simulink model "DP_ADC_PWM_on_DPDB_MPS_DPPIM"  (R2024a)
settings: Solver=FixedStepDiscrete  StartTime=0.0  StopTime=inf  FixedStep=10e-6  RelTol=1e-3  EnableMultiTasking=on
model workspace (MAT data in the model file):
  Freq = 100
  Phas = 0
undefined symbols (not defined in the file): a, A0, A2, A8, AD1, AD2, AD3, AD4, AD5, ADC, address, also, AN0, AN1, AN3, AN4, as, B, B0, B5, B6, B8, below, bit, bits, BOR, C6, C7, cause, characters, Code, Communicate, contains, counter, Data, data, dead, default, deviced, disasserted, DS70005399D, dsPIC33AK512MPS506_DPDB_External_v4, dsPIC33AK512MPS506_DPDB_External_v5, dsPIC33CK64MC105, EC, ECIO, ensure, events, Family, faster, Floating, fulll, highest, HS, HS3, I, I2C, I2C1, I2C2, I2C3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
libraries: MCHP_Blockset x10, simulink x1
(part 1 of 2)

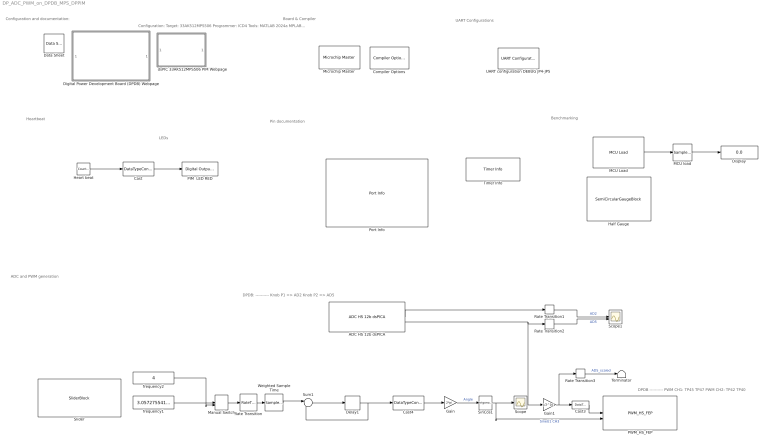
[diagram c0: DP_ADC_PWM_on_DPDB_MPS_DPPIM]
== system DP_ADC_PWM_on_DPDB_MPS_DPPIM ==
  note: DPDB: ---------- Knob P1 => AD2 Knob P2 => AD5
  note: Configuration and documentation:
  note: Configuration: Target: 33AK512MPS506 Programmer: ICD4 Tools: MATLAB 2024a MPLAB X 6.25 xc-dsc 3.21 DFP 1.2.135 MPLAB Blockset for Simulink 3.62
  note: Pin documentation
  note: Heartbeat
  note: Benchmarking
  note: ADC and PWM generation
  note: DPDB ---------- PWM CH1: TP45 TP47 PWM CH2: TP42 TP40
  note: UART Configurations
  note: LEDs
  note: Board & Compiler
  ADC HS 12b dsPICA : MCHP_Blockset/Analog IO/ADC HS 12b dsPICA  ADCREF=ADC 1 and ADC 2  ADC1_refChannel=Not used  ADC2_refChannel=0 (highest priority)  ADC3_refChannel=Not used  ADC4_refChannel=Not used  ADC5_refChannel=0 (highest priority)  CALRATE=once at startup  VREF_RNG=3.0V to 3.6V  BUFEN=on  info=0  SampleTime=10e-6  MCHP_PORT={ADC1_seq0.0}{ADC1A2}15:2:A2;{ADC2_seq0.0}{ADC2B8}15:2:B8;{ADC1_seq0.0}{ADC1A2}15:2:A2;{ADC2_seq0.0}{ADC2B8}15:2:B8;  MCHP_MASTERLINK=dsPIC33AK512MPS506_DPDB_External_v4/Microchip Master  MCHP_CRC=34143797  ADC_Synchronisation=Triggered at end of previous time step  ADC_Trig_TXT=Timer  ADC_TrigTimeStep=on  TrigSource_seq0=Dynamic Options  TrigSource_seq0_TXT=at end of previous time step  SampleTime_seq0_Tad=Dynamic Options  SampleTime_seq0_Tad_TXT="8.5 Tad  = 106ns  -  Rin < 11 kOhm"  ADC1_seq0=Dynamic Options  ADC1_seq0_TXT=AD1 AN0 / A2 / Pin[12]  ADC1_seq0_align=Left aligned  ADC1_seq0_overSampling=x1 (12 bits)  ADC2_seq0=Dynamic Options  ADC2_seq0_TXT=AD2 AN4 / B8 / Pin[23]  ADC2_seq0_align=Right aligned  ADC2_seq0_overSampling=x256 (16 bits)  ADC3_seq0=Dynamic Options  ADC3_seq0_TXT=AD3 AN1 / B5 / Pin[17]  ADC3_seq0_align=Right aligned  ADC3_seq0_overSampling=x256 (16 bits)  ADC4_seq0=Dynamic Options  ADC4_seq0_TXT=AD4 AN1 / B6 / Pin[29]  ADC4_seq0_align=Right aligned  ADC4_seq0_overSampling=x256 (16 bits)  ADC5_seq0=Dynamic Options  ADC5_seq0_TXT=AD5 AN3 / A8 / Pin[7]  ADC5_seq0_align=Right aligned  ADC5_seq0_overSampling=x256 (16 bits)  ADC1_seq0_1=Dynamic Options  ADC1_seq0_1_TXT=Not Used  ADC1_seq0_1_align=Right aligned  ADC1_seq0_1_overSampling=x1 (12 bits)  ADC2_seq0_1=Dynamic Options  ADC2_seq0_1_TXT=Not Used  ADC2_seq0_1_align=Right aligned  ADC2_seq0_1_overSampling=x1 (12 bits)  ADC3_seq0_1=Dynamic Options  ADC3_seq0_1_TXT=Not Used  ADC3_seq0_1_align=Right aligned  ADC3_seq0_1_overSampling=x1 (12 bits)  ADC4_seq0_1=Dynamic Options  ADC4_seq0_1_TXT=Not Used  ADC4_seq0_1_align=Right aligned  ADC4_seq0_1_overSampling=x1 (12 bits)  ADC5_seq0_1=Dynamic Options  ADC5_seq0_1_TXT=Not Used  ADC5_seq0_1_align=Right aligned  ADC5_seq0_1_overSampling=x1 (12 bits)  ADC1_seq0_2=Dynamic Options  ADC1_seq0_2_TXT=Not Used  ADC1_seq0_2_align=Right aligned  ADC1_seq0_2_overSampling=x1 (12 bits)  ADC2_seq0_2=Dynamic Options  ADC2_seq0_2_TXT=Not Used  ADC2_seq0_2_align=Right aligned  ADC2_seq0_2_overSampling=x1 (12 bits)  ADC3_seq0_2=Dynamic Options  ADC3_seq0_2_TXT=Not Used  ADC3_seq0_2_align=Right aligned  ADC3_seq0_2_overSampling=x1 (12 bits)  ADC4_seq0_2=Dynamic Options  ADC4_seq0_2_TXT=Not Used  ADC4_seq0_2_align=Right aligned  ADC4_seq0_2_overSampling=x1 (12 bits)  ADC5_seq0_2=Dynamic Options  ADC5_seq0_2_TXT=Not Used  ADC5_seq0_2_align=Right aligned  ADC5_seq0_2_overSampling=x1 (12 bits)  ADC1_seq0_3=Dynamic Options  ADC1_seq0_3_TXT=Not Used  ADC1_seq0_3_align=Right aligned  ADC1_seq0_3_overSampling=x1 (12 bits)  ADC2_seq0_3=Dynamic Options  ADC2_seq0_3_TXT=Not Used  ADC2_seq0_3_align=Right aligned  ADC2_seq0_3_overSampling=x1 (12 bits)  ADC3_seq0_3=Dynamic Options  ADC3_seq0_3_TXT=Not Used  ADC3_seq0_3_align=Right aligned  ADC3_seq0_3_overSampling=x1 (12 bits)  ADC4_seq0_3=Dynamic Options  ADC4_seq0_3_TXT=Not Used  ADC4_seq0_3_align=Right aligned  ADC4_seq0_3_overSampling=x1 (12 bits)  ADC5_seq0_3=Dynamic Options  ADC5_seq0_3_TXT=Not Used  ADC5_seq0_3_align=Right aligned  ADC5_seq0_3_overSampling=x1 (12 bits)  ADC1_seq0_4=Dynamic Options  ADC1_seq0_4_TXT=Not Used  ADC1_seq0_4_align=Right aligned  ADC1_seq0_4_overSampling=x1 (12 bits)  ADC2_seq0_4=Dynamic Options  ADC2_seq0_4_TXT=Not Used  ADC2_seq0_4_align=Right aligned  ADC2_seq0_4_overSampling=x1 (12 bits)  ADC3_seq0_4=Dynamic Options  ADC3_seq0_4_TXT=Not Used  ADC3_seq0_4_align=Right aligned  ADC3_seq0_4_overSampling=x1 (12 bits)  ADC4_seq0_4=Dynamic Options  ADC4_seq0_4_TXT=Not Used  ADC4_seq0_4_align=Right aligned  ADC4_seq0_4_overSampling=x1 (12 bits)  ADC5_seq0_4=Dynamic Options  ADC5_seq0_4_TXT=Not Used  ADC5_seq0_4_align=Right aligned  ADC5_seq0_4_overSampling=x1 (12 bits)  ADC1_seq0_5=Dynamic Options  ADC1_seq0_5_TXT=Not Used  ADC1_seq0_5_align=Right aligned  ADC1_seq0_5_overSampling=x1 (12 bits)  ADC2_seq0_5=Dynamic Options  ADC2_seq0_5_TXT=Not Used  ADC2_seq0_5_align=Right aligned  ADC2_seq0_5_overSampling=x1 (12 bits)  ADC3_seq0_5=Dynamic Options  ADC3_seq0_5_TXT=Not Used  ADC3_seq0_5_align=Right aligned  ADC3_seq0_5_overSampling=x1 (12 bits)  ADC4_seq0_5=Dynamic Options  ADC4_seq0_5_TXT=Not Used  ADC4_seq0_5_align=Right aligned  ADC4_seq0_5_overSampling=x1 (12 bits)  ADC5_seq0_5=Dynamic Options  ADC5_seq0_5_TXT=Not Used  ADC5_seq0_5_align=Right aligned  ADC5_seq0_5_overSampling=x1 (12 bits)  ADC_TRG2_ACCBRST_seq0=Burst - not interruptible  ADC1_NINSEL_seq0=Dynamic Options  ADC1_NINSEL_seq0_TXT=Vss - single ended (unsigned)  ADC2_NINSEL_seq0=Dynamic Options  ADC2_NINSEL_seq0_TXT=Vss - single ended (unsigned)  ADC3_NINSEL_seq0=Dynamic Options  ADC3_NINSEL_seq0_TXT=Vss - single ended (unsigned)  ADC4_NINSEL_seq0=Dynamic Options  ADC4_NINSEL_seq0_TXT=Vss - single ended (unsigned)  ADC5_NINSEL_seq0=Dynamic Options  ADC5_NINSEL_seq0_TXT=Vss - single ended (unsigned)  TrigTimeStep_seq0=on  info_seq0=0  TrigSource_seq1=Dynamic Options  TrigSource_seq1_TXT=after previous sequence  SampleTime_seq1_Tad=Dynamic Options  SampleTime_seq1_Tad_TXT="0.5 Tad  = 6.25ns  -  Rin < 0 kOhm"  ADC1_seq1=Dynamic Options  ADC1_seq1_TXT=Not Used  ADC1_seq1_align=Right aligned  ADC1_seq1_overSampling=x1 (12 bits)  ADC2_seq1=Dynamic Options  ADC2_seq1_TXT=Not Used  ADC2_seq1_align=Right aligned  ADC2_seq1_overSampling=x1 (12 bits)  ADC3_seq1=Dynamic Options  ADC3_seq1_TXT=Not Used  ADC3_seq1_align=Right aligned  ADC3_seq1_overSampling=x1 (12 bits)  ADC4_seq1=Dynamic Options  ADC4_seq1_TXT=Not Used  ADC4_seq1_align=Right aligned  ADC4_seq1_overSampling=x1 (12 bits)  ADC5_seq1=Dynamic Options  ADC5_seq1_TXT=Not Used  ADC5_seq1_align=Right aligned  ADC5_seq1_overSampling=x1 (12 bits)  ADC1_seq1_1=Dynamic Options  ADC1_seq1_1_TXT=Not Used  ADC1_seq1_1_align=Right aligned  ADC1_seq1_1_overSampling=x1 (12 bits)  ADC2_seq1_1=Dynamic Options  ADC2_seq1_1_TXT=Not Used  ADC2_seq1_1_align=Right aligned  ADC2_seq1_1_overSampling=x1 (12 bits)  ADC3_seq1_1=Dynamic Options  ADC3_seq1_1_TXT=Not Used  ADC3_seq1_1_align=Right aligned  ADC3_seq1_1_overSampling=x1 (12 bits)  ADC4_seq1_1=Dynamic Options  ADC4_seq1_1_TXT=Not Used  ADC4_seq1_1_align=Right aligned  ADC4_seq1_1_overSampling=x1 (12 bits)  ADC5_seq1_1=Dynamic Options  ADC5_seq1_1_TXT=Not Used  ADC5_seq1_1_align=Right aligned  ADC5_seq1_1_overSampling=x1 (12 bits)  ADC1_seq1_2=Dynamic Options  ADC1_seq1_2_TXT=Not Used  ADC1_seq1_2_align=Right aligned  ADC1_seq1_2_overSampling=x1 (12 bits)  ADC2_seq1_2=Dynamic Options  ADC2_seq1_2_TXT=Not Used  ADC2_seq1_2_align=Right aligned  ADC2_seq1_2_overSampling=x1 (12 bits)  ADC3_seq1_2=Dynamic Options  ADC3_seq1_2_TXT=Not Used  ADC3_seq1_2_align=Right aligned  ADC3_seq1_2_overSampling=x1 (12 bits)  ADC4_seq1_2=Dynamic Options  ADC4_seq1_2_TXT=Not Used  ADC4_seq1_2_align=Right aligned  ADC4_seq1_2_overSampling=x1 (12 bits)  ADC5_seq1_2=Dynamic Options  ADC5_seq1_2_TXT=Not Used  ADC5_seq1_2_align=Right aligned  ADC5_seq1_2_overSampling=x1 (12 bits)  ADC1_seq1_3=Dynamic Options  ADC1_seq1_3_TXT=Not Used  ADC1_seq1_3_align=Right aligned  ADC1_seq1_3_overSampling=x1 (12 bits)  ADC2_seq1_3=Dynamic Options  ADC2_seq1_3_TXT=Not Used  ADC2_seq1_3_align=Right aligned  ADC2_seq1_3_overSampling=x1 (12 bits)  ADC3_seq1_3=Dynamic Options  ADC3_seq1_3_TXT=Not Used  ADC3_seq1_3_align=Right aligned  ADC3_seq1_3_overSampling=x1 (12 bits)  ADC4_seq1_3=Dynamic Options  ADC4_seq1_3_TXT=Not Used  ADC4_seq1_3_align=Right aligned  ADC4_seq1_3_overSampling=x1 (12 bits)  ADC5_seq1_3=Dynamic Options  ADC5_seq1_3_TXT=Not Used  ADC5_seq1_3_align=Right aligned  ADC5_seq1_3_overSampling=x1 (12 bits)  ADC1_seq1_4=Dynamic Options  ADC1_seq1_4_TXT=Not Used  ADC1_seq1_4_align=Right aligned  ADC1_seq1_4_overSampling=x1 (12 bits)  ADC2_seq1_4=Dynamic Options  ADC2_seq1_4_TXT=Not Used  ADC2_seq1_4_align=Right aligned  ADC2_seq1_4_overSampling=x1 (12 bits)  ADC3_seq1_4=Dynamic Options  ADC3_seq1_4_TXT=Not Used  ADC3_seq1_4_align=Right aligned  ADC3_seq1_4_overSampling=x1 (12 bits)  ADC4_seq1_4=Dynamic Options  ADC4_seq1_4_TXT=Not Used  ADC4_seq1_4_align=Right aligned  ADC4_seq1_4_overSampling=x1 (12 bits)  ADC5_seq1_4=Dynamic Options  ADC5_seq1_4_TXT=Not Used  ADC5_seq1_4_align=Right aligned  ADC5_seq1_4_overSampling=x1 (12 bits)  ADC1_seq1_5=Dynamic Options  ADC1_seq1_5_TXT=Not Used  ADC1_seq1_5_align=Right aligned  ADC1_seq1_5_overSampling=x1 (12 bits)  ADC2_seq1_5=Dynamic Options  ADC2_seq1_5_TXT=Not Used  ADC2_seq1_5_align=Right aligned  ADC2_seq1_5_overSampling=x1 (12 bits)  ADC3_seq1_5=Dynamic Options  ADC3_seq1_5_TXT=Not Used  ADC3_seq1_5_align=Right aligned  ADC3_seq1_5_overSampling=x1 (12 bits)  ADC4_seq1_5=Dynamic Options  ADC4_seq1_5_TXT=Not Used  ADC4_seq1_5_align=Right aligned  ADC4_seq1_5_overSampling=x1 (12 bits)  ADC5_seq1_5=Dynamic Options  ADC5_seq1_5_TXT=Not Used  ADC5_seq1_5_align=Right aligned  ADC5_seq1_5_overSampling=x1 (12 bits)  ADC_TRG2_ACCBRST_seq1=Burst - not interruptible  ADC1_NINSEL_seq1=Dynamic Options  ADC1_NINSEL_seq1_TXT=Vss - single ended (unsigned)  ADC2_NINSEL_seq1=Dynamic Options  ADC2_NINSEL_seq1_TXT=Vss - single ended (unsigned)  ADC3_NINSEL_seq1=Dynamic Options  ADC3_NINSEL_seq1_TXT=Vss - single ended (unsigned)  ADC4_NINSEL_seq1=Dynamic Options  ADC4_NINSEL_seq1_TXT=Vss - single ended (unsigned)  ADC5_NINSEL_seq1=Dynamic Options  ADC5_NINSEL_seq1_TXT=Vss - single ended (unsigned)  TrigTimeStep_seq1=off  info_seq1=0  TrigSource_seq2=Dynamic Options  TrigSource_seq2_TXT=after previous sequence  SampleTime_seq2_Tad=Dynamic Options  SampleTime_seq2_Tad_TXT="0.5 Tad  = 6.25ns  -  Rin < 0 kOhm"  ADC1_seq2=Dynamic Options  ADC1_seq2_TXT=Not Used  ADC1_seq2_align=Right aligned  ADC1_seq2_overSampling=x1 (12 bits)  ADC2_seq2=Dynamic Options  ADC2_seq2_TXT=Not Used  ADC2_seq2_align=Right aligned  ADC2_seq2_overSampling=x1 (12 bits)  ADC3_seq2=Dynamic Options  ADC3_seq2_TXT=Not Used  ADC3_seq2_align=Right aligned  ADC3_seq2_overSampling=x1 (12 bits)  ADC4_seq2=Dynamic Options  ADC4_seq2_TXT=Not Used  ADC4_seq2_align=Right aligned  ADC4_seq2_overSampling=x1 (12 bits)  ADC5_seq2=Dynamic Options  ADC5_seq2_TXT=Not Used  ADC5_seq2_align=Right aligned  ADC5_seq2_overSampling=x1 (12 bits)  ADC1_seq2_1=Dynamic Options  ADC1_seq2_1_TXT=Not Used  ADC1_seq2_1_align=Right aligned  ADC1_seq2_1_overSampling=x1 (12 bits)  ADC2_seq2_1=Dynamic Options  ADC2_seq2_1_TXT=Not Used  ADC2_seq2_1_align=Right aligned  ADC2_seq2_1_overSampling=x1 (12 bits)  ADC3_seq2_1=Dynamic Options  ADC3_seq2_1_TXT=Not Used  ADC3_seq2_1_align=Right aligned  ADC3_seq2_1_overSampling=x1 (12 bits)  ADC4_seq2_1=Dynamic Options  ADC4_seq2_1_TXT=Not Used  ADC4_seq2_1_align=Right aligned  ADC4_seq2_1_overSampling=x1 (12 bits)  ADC5_seq2_1=Dynamic Options  ADC5_seq2_1_TXT=Not Used  ADC5_seq2_1_align=Right aligned  ADC5_seq2_1_overSampling=x1 (12 bits)  ADC1_seq2_2=Dynamic Options  ADC1_seq2_2_TXT=Not Used  ADC1_seq2_2_align=Right aligned  ADC1_seq2_2_overSampling=x1 (12 bits)  ADC2_seq2_2=Dynamic Options  ADC2_seq2_2_TXT=Not Used  ADC2_seq2_2_align=Right aligned  ADC2_seq2_2_overSampling=x1 (12 bits)  ADC3_seq2_2=Dynamic Options  ADC3_seq2_2_TXT=Not Used  ADC3_seq2_2_align=Right aligned  ADC3_seq2_2_overSampling=x1 (12 bits)  ADC4_seq2_2=Dynamic Options  ADC4_seq2_2_TXT=Not Used  ADC4_seq2_2_align=Right aligned  ADC4_seq2_2_overSampling=x1 (12 bits)  ADC5_seq2_2=Dynamic Options  ADC5_seq2_2_TXT=Not Used  ADC5_seq2_2_align=Right aligned  ADC5_seq2_2_overSampling=x1 (12 bits)  ADC1_seq2_3=Dynamic Options  ADC1_seq2_3_TXT=Not Used  ADC1_seq2_3_align=Right aligned  ADC1_seq2_3_overSampling=x1 (12 bits)  ADC2_seq2_3=Dynamic Options  ADC2_seq2_3_TXT=Not Used  ADC2_seq2_3_align=Right aligned  ADC2_seq2_3_overSampling=x1 (12 bits)  ADC3_seq2_3=Dynamic Options  ADC3_seq2_3_TXT=Not Used  ADC3_seq2_3_align=Right aligned  ADC3_seq2_3_overSampling=x1 (12 bits)  ADC4_seq2_3=Dynamic Options  ADC4_seq2_3_TXT=Not Used  ADC4_seq2_3_align=Right aligned  ADC4_seq2_3_overSampling=x1 (12 bits)  ADC5_seq2_3=Dynamic Options  ADC5_seq2_3_TXT=Not Used  ADC5_seq2_3_align=Right aligned  ADC5_seq2_3_overSampling=x1 (12 bits)  ADC1_seq2_4=Dynamic Options  ADC1_seq2_4_TXT=Not Used  ADC1_seq2_4_align=Right aligned  ADC1_seq2_4_overSampling=x1 (12 bits)  ADC2_seq2_4=Dynamic Options  ADC2_seq2_4_TXT=Not Used  ADC2_seq2_4_align=Right aligned  ADC2_seq2_4_overSampling=x1 (12 bits)  ADC3_seq2_4=Dynamic Options  ADC3_seq2_4_TXT=Not Used  ADC3_seq2_4_align=Right aligned  ADC3_seq2_4_overSampling=x1 (12 bits)  ADC4_seq2_4=Dynamic Options  ADC4_seq2_4_TXT=Not Used  ADC4_seq2_4_align=Right aligned  ADC4_seq2_4_overSampling=x1 (12 bits)  ADC5_seq2_4=Dynamic Options  ADC5_seq2_4_TXT=Not Used  ADC5_seq2_4_align=Right aligned  ADC5_seq2_4_overSampling=x1 (12 bits)  ADC1_seq2_5=Dynamic Options  ADC1_seq2_5_TXT=Not Used  ADC1_seq2_5_align=Right aligned  ADC1_seq2_5_overSampling=x1 (12 bits)  ADC2_seq2_5=Dynamic Options  ADC2_seq2_5_TXT=Not Used  ADC2_seq2_5_align=Right aligned  ADC2_seq2_5_overSampling=x1 (12 bits)  ADC3_seq2_5=Dynamic Options  ADC3_seq2_5_TXT=Not Used  ADC3_seq2_5_align=Right aligned  ADC3_seq2_5_overSampling=x1 (12 bits)  ADC4_seq2_5=Dynamic Options  ADC4_seq2_5_TXT=Not Used  ADC4_seq2_5_align=Right aligned  ADC4_seq2_5_overSampling=x1 (12 bits)  ADC5_seq2_5=Dynamic Options  ADC5_seq2_5_TXT=Not Used  ADC5_seq2_5_align=Right aligned  ADC5_seq2_5_overSampling=x1 (12 bits)  ADC_TRG2_ACCBRST_seq2=Burst - not interruptible  ADC1_NINSEL_seq2=Dynamic Options  ADC1_NINSEL_seq2_TXT=Vss - single ended (unsigned)  ADC2_NINSEL_seq2=Dynamic Options  ADC2_NINSEL_seq2_TXT=Vss - single ended (unsigned)  ADC3_NINSEL_seq2=Dynamic Options  ADC3_NINSEL_seq2_TXT=Vss - single ended (unsigned)  ADC4_NINSEL_seq2=Dynamic Options  ADC4_NINSEL_seq2_TXT=Vss - single ended (unsigned)  ADC5_NINSEL_seq2=Dynamic Options  ADC5_NINSEL_seq2_TXT=Vss - single ended (unsigned)  TrigTimeStep_seq2=off  info_seq2=0  TrigSource_seq3=Dynamic Options  TrigSource_seq3_TXT=after previous sequence  SampleTime_seq3_Tad=Dynamic Options  SampleTime_seq3_Tad_TXT="0.5 Tad  = 6.25ns  -  Rin < 0 kOhm"  ADC1_seq3=Dynamic Options  ADC1_seq3_TXT=Not Used  ADC1_seq3_align=Right aligned  ADC1_seq3_overSampling=x1 (12 bits)  ADC2_seq3=Dynamic Options  ADC2_seq3_TXT=Not Used  ADC2_seq3_align=Right aligned  ADC2_seq3_overSampling=x1 (12 bits)  ADC3_seq3=Dynamic Options  ADC3_seq3_TXT=Not Used  ADC3_seq3_align=Right aligned  ADC3_seq3_overSampling=x1 (12 bits)  ADC4_seq3=Dynamic Options  ADC4_seq3_TXT=Not Used  ADC4_seq3_align=Right aligned  ADC4_seq3_overSampling=x1 (12 bits)  ADC5_seq3=Dynamic Options  ADC5_seq3_TXT=Not Used  ADC5_seq3_align=Right aligned  ADC5_seq3_overSampling=x1 (12 bits)  ADC1_seq3_1=Dynamic Options  ADC1_seq3_1_TXT=Not Used  ADC1_seq3_1_align=Right aligned  ADC1_seq3_1_overSampling=x1 (12 bits)  ADC2_seq3_1=Dynamic Options  ADC2_seq3_1_TXT=Not Used  ADC2_seq3_1_align=Right aligned  ADC2_seq3_1_overSampling=x1 (12 bits)  ADC3_seq3_1=Dynamic Options  ADC3_seq3_1_TXT=Not Used  ADC3_seq3_1_align=Right aligned  ADC3_seq3_1_overSampling=x1 (12 bits)  ADC4_seq3_1=Dynamic Options  ADC4_seq3_1_TXT=Not Used  ADC4_seq3_1_align=Right aligned  ADC4_seq3_1_overSampling=x1 (12 bits)  ADC5_seq3_1=Dynamic Options  ADC5_seq3_1_TXT=Not Used  ADC5_seq3_1_align=Right aligned  ADC5_seq3_1_overSampling=x1 (12 bits)  ADC1_seq3_2=Dynamic Options  ADC1_seq3_2_TXT=Not Used  ADC1_seq3_2_align=Right aligned  ADC1_seq3_2_overSampling=x1 (12 bits)  ADC2_seq3_2=Dynamic Options  ADC2_seq3_2_TXT=Not Used  ADC2_seq3_2_align=Right aligned  ADC2_seq3_2_overSampling=x1 (12 bits)  ADC3_seq3_2=Dynamic Options  ADC3_seq3_2_TXT=Not Used  ADC3_seq3_2_align=Right aligned  ADC3_seq3_2_overSampling=x1 (12 bits)  ADC4_seq3_2=Dynamic Options  ADC4_seq3_2_TXT=Not Used  ADC4_seq3_2_align=Right aligned  ADC4_seq3_2_overSampling=x1 (12 bits)  ADC5_seq3_2=Dynamic Options  ADC5_seq3_2_TXT=Not Used  ADC5_seq3_2_align=Right aligned  ADC5_seq3_2_overSampling=x1 (12 bits)  ADC1_seq3_3=Dynamic Options  ADC1_seq3_3_TXT=Not Used  ADC1_seq3_3_align=Right aligned  ADC1_seq3_3_overSampling=x1 (12 bits)  ADC2_seq3_3=Dynamic Options  ADC2_seq3_3_TXT=Not Used  ADC2_seq3_3_align=Right aligned  ADC2_seq3_3_overSampling=x1 (12 bits)  ADC3_seq3_3=Dynamic Options  ADC3_seq3_3_TXT=Not Used  ADC3_seq3_3_align=Right aligned  ADC3_seq3_3_overSampling=x1 (12 bits)  ADC4_seq3_3=Dynamic Options  ADC4_seq3_3_TXT=Not Used  ADC4_seq3_3_align=Right aligned  ADC4_seq3_3_overSampling=x1 (12 bits)  ADC5_seq3_3=Dynamic Options  ADC5_seq3_3_TXT=Not Used  ADC5_seq3_3_align=Right aligned  ADC5_seq3_3_overSampling=x1 (12 bits)  ADC1_seq3_4=Dynamic Options  ADC1_seq3_4_TXT=Not Used  ADC1_seq3_4_align=Right aligned  ADC1_seq3_4_overSampling=x1 (12 bits)  ADC2_seq3_4=Dynamic Options  ADC2_seq3_4_TXT=Not Used  ADC2_seq3_4_align=Right aligned  ADC2_seq3_4_overSampling=x1 (12 bits)  ADC3_seq3_4=Dynamic Options  ADC3_seq3_4_TXT=Not Used  ADC3_seq3_4_align=Right aligned  ADC3_seq3_4_overSampling=x1 (12 bits)  ADC4_seq3_4=Dynamic Options  ADC4_seq3_4_TXT=Not Used  ADC4_seq3_4_align=Right aligned  ADC4_seq3_4_overSampling=x1 (12 bits)  ADC5_seq3_4=Dynamic Options  ADC5_seq3_4_TXT=Not Used  ADC5_seq3_4_align=Right aligned  ADC5_seq3_4_overSampling=x1 (12 bits)  ADC1_seq3_5=Dynamic Options  ADC1_seq3_5_TXT=Not Used  ADC1_seq3_5_align=Right aligned  ADC1_seq3_5_overSampling=x1 (12 bits)  ADC2_seq3_5=Dynamic Options  ADC2_seq3_5_TXT=Not Used  ADC2_seq3_5_align=Right aligned  ADC2_seq3_5_overSampling=x1 (12 bits)  ADC3_seq3_5=Dynamic Options  ADC3_seq3_5_TXT=Not Used  ADC3_seq3_5_align=Right aligned  ADC3_seq3_5_overSampling=x1 (12 bits)  ADC4_seq3_5=Dynamic Options  ADC4_seq3_5_TXT=Not Used  ADC4_seq3_5_align=Right aligned  ADC4_seq3_5_overSampling=x1 (12 bits)  ADC5_seq3_5=Dynamic Options  ADC5_seq3_5_TXT=Not Used  ADC5_seq3_5_align=Right aligned  ADC5_seq3_5_overSampling=x1 (12 bits)  ADC_TRG2_ACCBRST_seq3=Burst - not interruptible  ADC1_NINSEL_seq3=Dynamic Options  ADC1_NINSEL_seq3_TXT=Vss - single ended (unsigned)  ADC2_NINSEL_seq3=Dynamic Options  ADC2_NINSEL_seq3_TXT=Vss - single ended (unsigned)  ADC3_NINSEL_seq3=Dynamic Options  ADC3_NINSEL_seq3_TXT=Vss - single ended (unsigned)  ADC4_NINSEL_seq3=Dynamic Options  ADC4_NINSEL_seq3_TXT=Vss - single ended (unsigned)  ADC5_NINSEL_seq3=Dynamic Options  ADC5_NINSEL_seq3_TXT=Vss - single ended (unsigned)  TrigTimeStep_seq3=off  info_seq3=0  TrigSource_seq4=Dynamic Options  TrigSource_seq4_TXT=after previous sequence  SampleTime_seq4_Tad=Dynamic Options  SampleTime_seq4_Tad_TXT="0.5 Tad  = 6.25ns  -  Rin < 0 kOhm"  ADC1_seq4=Dynamic Options  ADC1_seq4_TXT=Not Used  ADC1_seq4_align=Right aligned  ADC1_seq4_overSampling=x1 (12 bits)  ADC2_seq4=Dynamic Options  ADC2_seq4_TXT=Not Used  ADC2_seq4_align=Right aligned  ADC2_seq4_overSampling=x1 (12 bits)  ADC3_seq4=Dynamic Options  ADC3_seq4_TXT=Not Used  ADC3_seq4_align=Right aligned  ADC3_seq4_overSampling=x1 (12 bits)  ADC4_seq4=Dynamic Options  ADC4_seq4_TXT=Not Used  ADC4_seq4_align=Right aligned  ADC4_seq4_overSampling=x1 (12 bits)  ADC5_seq4=Dynamic Options  ADC5_seq4_TXT=Not Used  ADC5_seq4_align=Right aligned  ADC5_seq4_overSampling=x1 (12 bits)  ADC1_seq4_1=Dynamic Options  ADC1_seq4_1_TXT=Not Used  ADC1_seq4_1_align=Right aligned  ADC1_seq4_1_overSampling=x1 (12 bits)  ADC2_seq4_1=Dynamic Options  ADC2_seq4_1_TXT=Not Used  ADC2_seq4_1_align=Right aligned  ADC2_seq4_1_overSampling=x1 (12 bits)  ADC3_seq4_1=Dynamic Options  ADC3_seq4_1_TXT=Not Used  ADC3_seq4_1_align=Right aligned  ADC3_seq4_1_overSampling=x1 (12 bits)  ADC4_seq4_1=Dynamic Options  ADC4_seq4_1_TXT=Not Used  ADC4_seq4_1_align=Right aligned  ADC4_seq4_1_overSampling=x1 (12 bits)  ADC5_seq4_1=Dynamic Options  ADC5_seq4_1_TXT=Not Used  ADC5_seq4_1_align=Right aligned  ADC5_seq4_1_overSampling=x1 (12 bits)  ADC1_seq4_2=Dynamic Options  ADC1_seq4_2_TXT=Not Used  ADC1_seq4_2_align=Right aligned  ADC1_seq4_2_overSampling=x1 (12 bits)  ADC2_seq4_2=Dynamic Options  ADC2_seq4_2_TXT=Not Used  ADC2_seq4_2_align=Right aligned  ADC2_seq4_2_overSampling=x1 (12 bits)  ADC3_seq4_2=Dynamic Options  ADC3_seq4_2_TXT=Not Used  ADC3_seq4_2_align=Right aligned  ADC3_seq4_2_overSampling=x1 (12 bits)  ADC4_seq4_2=Dynamic Options  ADC4_seq4_2_TXT=Not Used  ADC4_seq4_2_align=Right aligned  ADC4_seq4_2_overSampling=x1 (12 bits)  ADC5_seq4_2=Dynamic Options  ADC5_seq4_2_TXT=Not Used  ADC5_seq4_2_align=Right aligned  ADC5_seq4_2_overSampling=x1 (12 bits)  ADC1_seq4_3=Dynamic Options  ADC1_seq4_3_TXT=Not Used  ADC1_seq4_3_align=Right aligned  ADC1_seq4_3_overSampling=x1 (12 bits)  ADC2_seq4_3=Dynamic Options  ADC2_seq4_3_TXT=Not Used  ADC2_seq4_3_align=Right aligned  ADC2_seq4_3_overSampling=x1 (12 bits)  ADC3_seq4_3=Dynamic Options  ADC3_seq4_3_TXT=Not Used  ADC3_seq4_3_align=Right aligned  ADC3_seq4_3_overSampling=x1 (12 bits)  ADC4_seq4_3=Dynamic Options  ADC4_seq4_3_TXT=Not Used  ADC4_seq4_3_align=Right aligned  ADC4_seq4_3_overSampling=x1 (12 bits)  ADC5_seq4_3=Dynamic Options  ADC5_seq4_3_TXT=Not Used  ADC5_seq4_3_align=Right aligned  ADC5_seq4_3_overSampling=x1 (12 bits)  ADC1_seq4_4=Dynamic Options  ADC1_seq4_4_TXT=Not Used  ADC1_seq4_4_align=Right aligned  ADC1_seq4_4_overSampling=x1 (12 bits)  ADC2_seq4_4=Dynamic Options  ADC2_seq4_4_TXT=Not Used  ADC2_seq4_4_align=Right aligned  ADC2_seq4_4_overSampling=x1 (12 bits)  ADC3_seq4_4=Dynamic Options  ADC3_seq4_4_TXT=Not Used  ADC3_seq4_4_align=Right aligned  ADC3_seq4_4_overSampling=x1 (12 bits)  ADC4_seq4_4=Dynamic Options  ADC4_seq4_4_TXT=Not Used  ADC4_seq4_4_align=Right aligned  ADC4_seq4_4_overSampling=x1 (12 bits)  ADC5_seq4_4=Dynamic Options  ADC5_seq4_4_TXT=Not Used  ADC5_seq4_4_align=Right aligned  ADC5_seq4_4_overSampling=x1 (12 bits)  ADC1_seq4_5=Dynamic Options  ADC1_seq4_5_TXT=Not Used  ADC1_seq4_5_align=Right aligned  ADC1_seq4_5_overSampling=x1 (12 bits)  ADC2_seq4_5=Dynamic Options  ADC2_seq4_5_TXT=Not Used  ADC2_seq4_5_align=Right aligned  ADC2_seq4_5_overSampling=x1 (12 bits)  ADC3_seq4_5=Dynamic Options  ADC3_seq4_5_TXT=Not Used  ADC3_seq4_5_align=Right aligned  ADC3_seq4_5_overSampling=x1 (12 bits)  ADC4_seq4_5=Dynamic Options  ADC4_seq4_5_TXT=Not Used  ADC4_seq4_5_align=Right aligned  ADC4_seq4_5_overSampling=x1 (12 bits)  ADC5_seq4_5=Dynamic Options  ADC5_seq4_5_TXT=Not Used  ADC5_seq4_5_align=Right aligned  ADC5_seq4_5_overSampling=x1 (12 bits)  ADC_TRG2_ACCBRST_seq4=Burst - not interruptible  ADC1_NINSEL_seq4=Dynamic Options  ADC1_NINSEL_seq4_TXT=Vss - single ended (unsigned)  ADC2_NINSEL_seq4=Dynamic Options  ADC2_NINSEL_seq4_TXT=Vss - single ended (unsigned)  ADC3_NINSEL_seq4=Dynamic Options  ADC3_NINSEL_seq4_TXT=Vss - single ended (unsigned)  ADC4_NINSEL_seq4=Dynamic Options  ADC4_NINSEL_seq4_TXT=Vss - single ended (unsigned)  ADC5_NINSEL_seq4=Dynamic Options  ADC5_NINSEL_seq4_TXT=Vss - single ended (unsigned)  TrigTimeStep_seq4=off  info_seq4=0  TrigSource_seq5=Dynamic Options  TrigSource_seq5_TXT=after previous sequence  SampleTime_seq5_Tad=Dynamic Options  SampleTime_seq5_Tad_TXT="0.5 Tad  = 6.25ns  -  Rin < 0 kOhm"  ADC1_seq5=Dynamic Options  ADC1_seq5_TXT=Not Used  ADC1_seq5_align=Right aligned  ADC1_seq5_overSampling=x1 (12 bits)  ADC2_seq5=Dynamic Options  ADC2_seq5_TXT=Not Used  ADC2_seq5_align=Right aligned  ADC2_seq5_overSampling=x1 (12 bits)  ADC3_seq5=Dynamic Options  ADC3_seq5_TXT=Not Used  ADC3_seq5_align=Right aligned  ADC3_seq5_overSampling=x1 (12 bits)  ADC4_seq5=Dynamic Options  ADC4_seq5_TXT=Not Used  ADC4_seq5_align=Right aligned  ADC4_seq5_overSampling=x1 (12 bits)  ADC5_seq5=Dynamic Options  ADC5_seq5_TXT=Not Used  ADC5_seq5_align=Right aligned  ADC5_seq5_overSampling=x1 (12 bits)  ADC1_seq5_1=Dynamic Options  ADC1_seq5_1_TXT=Not Used  ADC1_seq5_1_align=Right aligned  ADC1_seq5_1_overSampling=x1 (12 bits)  ADC2_seq5_1=Dynamic Options  ADC2_seq5_1_TXT=Not Used  ADC2_seq5_1_align=Right aligned  ADC2_seq5_1_overSampling=x1 (12 bits)  ADC3_seq5_1=Dynamic Options  ADC3_seq5_1_TXT=Not Used  ADC3_seq5_1_align=Right aligned  ADC3_seq5_1_overSampling=x1 (12 bits)  ADC4_seq5_1=Dynamic Options  ADC4_seq5_1_TXT=Not Used  ADC4_seq5_1_align=Right aligned  ADC4_seq5_1_overSampling=x1 (12 bits)  ADC5_seq5_1=Dynamic Options  ADC5_seq5_1_TXT=Not Used  ADC5_seq5_1_align=Right aligned  ADC5_seq5_1_overSampling=x1 (12 bits)  ADC1_seq5_2=Dynamic Options  ADC1_seq5_2_TXT=Not Used  ADC1_seq5_2_align=Right aligned  ADC1_seq5_2_overSampling=x1 (12 bits)  ADC2_seq5_2=Dynamic Options  ADC2_seq5_2_TXT=Not Used  ADC2_seq5_2_align=Right aligned  ADC2_seq5_2_overSampling=x1 (12 bits)  ADC3_seq5_2=Dynamic Options  ADC3_seq5_2_TXT=Not Used  ADC3_seq5_2_align=Right aligned  ADC3_seq5_2_overSampling=x1 (12 bits)  ADC4_seq5_2=Dynamic Options  ADC4_seq5_2_TXT=Not Used  ADC4_seq5_2_align=Right aligned  ADC4_seq5_2_overSampling=x1 (12 bits)  ADC5_seq5_2=Dynamic Options  ADC5_seq5_2_TXT=Not Used  ADC5_seq5_2_align=Right aligned  ADC5_seq5_2_overSampling=x1 (12 bits)  ADC1_seq5_3=Dynamic Options  ADC1_seq5_3_TXT=Not Used  ADC1_seq5_3_align=Right aligned  ADC1_seq5_3_overSampling=x1 (12 bits)  ADC2_seq5_3=Dynamic Options  ADC2_seq5_3_TXT=Not Used  ADC2_seq5_3_align=Right aligned  ADC2_seq5_3_overSampling=x1 (12 bits)  ADC3_seq5_3=Dynamic Options  ADC3_seq5_3_TXT=Not Used  ADC3_seq5_3_align=Right aligned  ADC3_seq5_3_overSampling=x1 (12 bits)  ADC4_seq5_3=Dynamic Options  ADC4_seq5_3_TXT=Not Used  ADC4_seq5_3_align=Right aligned  ADC4_seq5_3_overSampling=x1 (12 bits)  ADC5_seq5_3=Dynamic Options  ADC5_seq5_3_TXT=Not Used  ADC5_seq5_3_align=Right aligned  ADC5_seq5_3_overSampling=x1 (12 bits)  ADC1_seq5_4=Dynamic Options  ADC1_seq5_4_TXT=Not Used  ADC1_seq5_4_align=Right aligned  ADC1_seq5_4_overSampling=x1 (12 bits)  ADC2_seq5_4=Dynamic Options  ADC2_seq5_4_TXT=Not Used  ADC2_seq5_4_align=Right aligned  ADC2_seq5_4_overSampling=x1 (12 bits)  ADC3_seq5_4=Dynamic Options  ADC3_seq5_4_TXT=Not Used  ADC3_seq5_4_align=Right aligned  ADC3_seq5_4_overSampling=x1 (12 bits)  ADC4_seq5_4=Dynamic Options  ADC4_seq5_4_TXT=Not Used  ADC4_seq5_4_align=Right aligned  ADC4_seq5_4_overSampling=x1 (12 bits)  ADC5_seq5_4=Dynamic Options  ADC5_seq5_4_TXT=Not Used  ADC5_seq5_4_align=Right aligned  ADC5_seq5_4_overSampling=x1 (12 bits)  ADC1_seq5_5=Dynamic Options  ADC1_seq5_5_TXT=Not Used  ADC1_seq5_5_align=Right aligned  ADC1_seq5_5_overSampling=x1 (12 bits)  ADC2_seq5_5=Dynamic Options  ADC2_seq5_5_TXT=Not Used  ADC2_seq5_5_align=Right aligned  ADC2_seq5_5_overSampling=x1 (12 bits)  ADC3_seq5_5=Dynamic Options  ADC3_seq5_5_TXT=Not Used  ADC3_seq5_5_align=Right aligned  ADC3_seq5_5_overSampling=x1 (12 bits)  ADC4_seq5_5=Dynamic Options  ADC4_seq5_5_TXT=Not Used  ADC4_seq5_5_align=Right aligned  ADC4_seq5_5_overSampling=x1 (12 bits)  ADC5_seq5_5=Dynamic Options  ADC5_seq5_5_TXT=Not Used  ADC5_seq5_5_align=Right aligned  ADC5_seq5_5_overSampling=x1 (12 bits)  ADC_TRG2_ACCBRST_seq5=Burst - not interruptible  ADC1_NINSEL_seq5=Dynamic Options  ADC1_NINSEL_seq5_TXT=Vss - single ended (unsigned)  ADC2_NINSEL_seq5=Dynamic Options  ADC2_NINSEL_seq5_TXT=Vss - single ended (unsigned)  ADC3_NINSEL_seq5=Dynamic Options  ADC3_NINSEL_seq5_TXT=Vss - single ended (unsigned)  ADC4_NINSEL_seq5=Dynamic Options  ADC4_NINSEL_seq5_TXT=Vss - single ended (unsigned)  ADC5_NINSEL_seq5=Dynamic Options  ADC5_NINSEL_seq5_TXT=Vss - single ended (unsigned)  TrigTimeStep_seq5=off  info_seq5=0
  Cast : DataTypeConversion
  Cast3 : DataTypeConversion  OutDataTypeStr=single
  Cast4 : DataTypeConversion  OutDataTypeStr=single
  Compiler Options : MCHP_Blockset/System Configuration/Compiler Options  Priority=1  LATEST_CMPLR=off  COMP_LIST=Dynamic Options  COMP_LIST_TXT=XC-DSC - v3.21  DFP_LIST=Dynamic Options  DFP_LIST_TXT=v 1.2.135  CMSIS_DSP=Dynamic Options  CMSIS_DSP_TXT=Dynamic Options  USE_64BIT_DOUBLE=on  MCHP_MULTITHREAD_COMPILATION=on  UseCustom_LinkerScript=off  MCHP_MASTERLINK=dsPIC33AK512MPS506_DPDB_External_v4/Microchip Master  OPTIMIZATION_LEVEL=2  MPLAB_LINKLIB=default  MPLAB_LINKLIB1=default  CodeReplacement=Dynamic Options  CodeReplacement_TXT=None  OPTIMIZATION_FLTO=on  OPTIMIZATION_REORDER=off  OPTIMIZATION_ASM_REORDER=on  UNROLL_LOOPS=off  PROCEDURAL_ABSTRACTION=off  CONSERVE_STACK=off  GC_SECTIONS=None  MCODE=is less than 32768 (faster)  MCONST=in code memory  MDATA=Can use all available memory  MSCALAR=Use only memory below address 8192 (faster)  MLARGEARRAY=off  MAGGREGATE=on  HEAP_SIZE=0  OMF=elf  DEBUG_INFO=on  MCHP_STACK_USAGE=off  GCC_STACK_USAGE=off  ProduceHexOutput=off  AssemblyListing=off  SaveTemps=off  NO_EDS_WARN=on  PRINT_STATISTICS=off
  Data Sheet : MCHP_Blockset/System Info/Data Sheet  DOC_Type=datasheet  DOC_MCHP_Id=33CK64MC105_datasheet  DOC_FilePath=/tmp/dsPIC33CK64MC105-Family-Data-Sheet-DS70005399D.pdf  DOC_FileLastCheckTime="[2023              3             13              0             36       3.057334]"  cpy_MCHP_Id=33AK512MPS506  MCHP_MASTERLINK=dsPIC33AK512MPS506_DPDB_External_v4/Microchip Master
  Delay1 : Delay  DelayLength=1  InitialCondition=0
  Digital Power Development Board (DPDB) Webpage : Subsystem
  Display : Display
  Gain : Gain  Gain=2*pi  ParamDataTypeStr=single  OutDataTypeStr=single
  Gain1 : Gain  Gain=1/2^16
  Half Gauge : SemiCircularGaugeBlock  ScaleMax=1
  Heart beat : simulink/Sources/Counter Free-Running  NumBits=1  tsamp=.25
  MCU Load : MCHP_Blockset/Profiling/MCU Load  MCULoadPin=Dynamic Options  MCULoadPin_TXT=A0 / Pin[1]  MCULoadMeasure=on  TIMER_Resolution=Dynamic Options  TIMER_Resolution_TXT="Resol: 0.04(us)  -  Max: 2.62(ms)"  MCHP_PORT={MCU Load Pin}{MCU_Load}0:1:A0;  MCHP_TIMER_REQUEST={MCU_Load}{MCU_Load}21:5:0:0:[]:131072;  MCHP_TIMER_RESULT=[5 65535 ]  MCHP_MASTERLINK=dsPIC33AK512MPS506_DPDB_External_v4/Microchip Master  MCHP_COMPILED_INFO="CompiledSampleTime= [0.0050000000000000001041   0 ];CompiledInportDataTypes=[    ];CompiledInportDataWidth=[];"  Info="Timer 5:  Resol: 20(ns)  -  Max: 1.31072(ms)"  SampleTime=.005
  MCU load : SampleTimeMath  TsampMathOp=/  weightValue=inv(40e-9)  OutDataTypeStr=fixdt(0,16,15)  RndMeth=Round  SaturateOnIntegerOverflow=on
  Manual Switch : ManualSwitch  CurrentSetting=0
  Microchip Master : MCHP_Blockset/System Configuration/Microchip Master  Priority=1  PICREF=33AK512MPS506  TIMESTEP_REF="Timer + ADC  ( 1e-05s )"  BUSYFLAG=Dynamic Options  BUSYFLAG_TXT=None  VDD_range=Dynamic Options  PWRTEN=Not used  BOREN=Disable  BODENV=2.7V  BORV=Not used  FPWRT=128ms  DSBOREN=Enable ZPBOR during Deep Sleep Mode  DSLPBOR=Not used  MCLRE=Enabled  SMCLR=MCLR pin generates a normal system Reset  PMDL1WAY=Allow only one reconfiguration  RSTPRI=Device will obtain reset instruction from Primary flash  TEMP=Not used  SOSCSRC=Not used  SOSCSEL=Not used  IOL1WAY=Allow only one reconfiguration  ALTVREF=Not used  DISUVREG=Not used  DSSWEN=Not used  LPCFG=Not used  RTCBAT=Not used  VBTBOR=Not used  WUTSEL=Not used  POWERSAVE=off  FNOSC=Primary Oscillator (XT; HS; EC)  FPR=ECIO w/ PLL 16x  FOSFPR=HS3 w/PLL 16x  FOS=Primary Oscillator  FRANGE=High Range  OSCILLATOR_SELECT=External Clock  OSCILLATOR_SELECT_spd=External Clock  QUARTZ=8e6  QUARTZ_spd=8e6  POSCGAIN=2x gain setting  POSCBOOST=Boost the kick start of the oscillator  SOSCGAIN=2x gain setting  SOSCBOOST=Boost the kick start of the oscillator  ACTIV_PLL=on  ACTIV_PLL_spd=on  MIPS_DESIRED=200e6  MIPS_DESIRED_spd=200e6  CPUDIV=Divide by 1  FPLLMUL=Not used  FPLLIDIV=8x Divider  POSCFREQ=Not used  POSCMD=EC (External Clock) Mode  POSCMOD=Primary Oscillator Disabled  MIPS=200 * 1e6  ACLKCON=Optimized for PWM resolution & ADC conversion speed  ACLKCON_spd=Optimized for PWM resolution & ADC conversion speed  FPLLODIV=32x Divider  PLLKEN=PLL lock signal will be used to disable PLL clock output if lock is lost  FCKSM=Both Clock switching and Fail-safe Clock Monitor are enabled  FCKSMEN=Sw Disabled; Mon Disabled  IESO=Start up with FRC; then switch  DSWDTPS=1:2^36  FWDTEN=WDT controlled via SW; use WDTCON.ON bit  FWDTWINSZ=Window size is 25%  FWPSA=1:512  FWPSA0=1:128  FWPSB=1:16  WDT=Disable  WDTPOST=1:32768  WDTPRE=1:128  WDTPS=1:32768  WINDIS=Watchdog Timer operates in Non-Window mode  WWDTEN=Non-Window mode  DSWDTEN=Enable DSWDT during Deep Sleep Mode  DSWDTOSC=Select LPRC as DSWDT Reference clock  FWDT_RCLKSEL=WDT Run Mode uses BFRC:256  FWDT_RWDTPS=1:2147483648  FWDT_SWDTMPS=1:2147483648  FWDT_WDTEN=WDT is controlled by software; use WDTCON.ON bit  FWDT_WDTRSTEN=WDT event generates a reset  FWDT_WDTWIN=WDT Window is 25% of WDT period  FWDT_WINEN=Watchdog Timer operates in Window mode  FPBDIV=Not used  FSOSCEN=Disable Secondary Oscillator  LPRCSEL=Not used  OSCIOFCN=Not used  OSCIOFNC=general purpose digital I/O pin  LVRCFG=Not used  PLL_96MHZ=Not used  PLL96MHZ=Not used  PLLDIV=Not used  WDTCLK=Not used  WDTCMX=Not used  WDTWIN=WDT Window is 25% of WDT period  XTCFG=24-32 MHz crystals  XTBST=Boost the kick-start  APL=Aux Flash Code protect is disabled  APLK=Aux Flash Write Protection or Code Protection is Enabled  AWRP=Auxiliary program memory is not write-protected  BSS=No Protection (other than BWRP)  BWP=Not used  BWRP=Boot Segment may be written  CP=Protection Disabled  EBS=No Boot EEPROM  ESS=No Segment Data EEPROM  GCP=General Segment Code protect is Disabled  GSS=No Protection (other than GWRP)  GSS0=Not used  GSSK=General Segment Write Protection or Code Protection is Enabled  GWRP=General Segment may be written  PWP=Not used  RBS=No Boot RAM  RSS=No Secure RAM  SSS=No Secure Segment  SWRP=Secure segment may be written  WPCFG=Not used  WPDIS=Not used  WPEND=Not used  WPFP=Not used  ICESEL=Communicate on PGEC1/PGED1  ICS=Communicate on PGC2 and PGD2  JTAGEN=Disable  FICD_JTAGEN=Disable  COE=Not used  RES=Not used  DEBUG=Debugger is disabled  BACKBUG=Not used  BKBUG=Not used  ALTI2C=I2C mapped to SDA1/SCL1 pins  ALTI2C1=I2C1 mapped to SDA1/SCL1 pins  ALTI2C2=I2C2 mapped to SDA2/SCL2 pins  ALTI2C3=I2C3 mapped to SDA3/SCL3 pins  FDEVOPT1_ALTI2C1=Not used  FDEVOPT1_ALTI2C2=Not used  FDEVOPT1_SPI2MAPDIS=Not used  FDEVOPT_ALTI2C1=Primary I2C1 pins are used  FDEVOPT_ALTI2C2=Primary I2C2 pins are used  FDEVOPT_ALTI2C3=Primary I2C3 pins are used  FDEVOPT_SPI2PIN=SPI2 pins are selected by peripheral pin selection feature  ALTQIO=QEA1; QEB1; INDX1 are selected as inputs to QEI1  ALTSS1=SS1A is selected as the I/O pin for SPI1  CMPPOL0=Hysteresis is applied to falling edge  CMPPOL1=Hysteresis is applied to falling edge  FCANIO=Not used  FETHIO=Default Ethernet I/O  FMIIEN=MII Enabled  FSRSSEL=Not used  FUSBIDIO=Controlled by the USB Module  FVBUSONIO=Not used  HPOL=PWM module high side output pins have active-high output polarity  HYST0=45 mV Hysteresis  HYST1=45 mV Hysteresis  I2C1SEL=Not used  LPOL=PWM module low side output pins have active-high output polarity  PWMPIN=PWM module pins controlled by PORT register at device Reset  RTCOSC=Not used  UPLLEN=USB PLL Disabled  UPLLIDIV=Not used  ATMOD8=Not used  ALTPMP=Not used  I2C2SEL=Not used  ALTADREF=Not used  ALTCVREF=Not used  PWMLOCK=PWM registers may be written without key sequence  INT_PRIORITY_DMA=0  MCHP_TIMER_REQUEST="{Time Step}{TS}0:2:3:1:[4   5   6   7   8   9  10  11  12]:1000;"  MCHP_TIMER_RESULT=[4 1999 ]  MCHP_PLLRegisters="[0        -1     16386        -1  16815713]"  MCHPVAR=MCHP.fcy.MIPS=2e+08;MCHP.fcy.SYSCLK=2e+08;MCHP.fcy.Fplli=8000000;MCHP.fcy.Fvco=1.2e+09;MCHP.fcy.Fpllo=2e+08;MCHP.fcy.PWM=2e+08;MCHP.fcy.ADC=80000000;MCHP.fcy.UART=2e+08;MCHP.fcy.SPI=2e+08;MCHP.fcy.BiSS=2e+08;MCHP.fcy.SCC=2e+08;MCHP.fcy.Timers=1e+08;MCHP.fcy.I2C=2e+08;MCHP.PowerSave=0;MCHP.TimeStepFactor=1;MCHP.TimeStep_Timer=4;MCHP.NTIMERS=3;MCHP.id.name='33AK512MPS506';MCHP.id.N=reshape([33 512 5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  MCHP_CRC=18397476  BTMODE=Device is in Single Boot (legacy) mode  RES1=Not used  PLLSS=Not used  RES2=Not used  ALTCMPI=Not used  BOREN1=Not used  ALTRB6=Not used  RETCFG=Not used  DFMCY=Not used  BSS2=No Boot Segment  BSEN=No Boot Segment  CWRP=Configuration Segment may be written  CSS=No Protection (other than CWRP)  AIVTDIS=Disabled AIVT  BSLIM=Not used  WDTEN=Disable  BTSWP=BOOTSWP instruction is disabled  DBCC=No Cross Connection between DAC outputs  CTXT1=Not Assigned  CTXT2=Not Assigned  SEQNUM=Not used  nSEQNUM=Not used  BOREN0=Enabled  DMTIVT=Not used  DMTCNT=2^31 (2147483648)  DMTEN=Dead Man Timer is Disabled and can be enabled by software  ON=Not used  USERID=Not used  RESERVED1=Not used  PGL1WAY=Allow only one reconfiguration  FPLLRNG=34-68 MHz Input  FPLLICLK=FRC is input to the System PLL  FPLLMULT=PLL Multiply by 128  UPLLFSEL=USB PLL input is 24 MHz  DMTINTV=Window/Interval value is 127/128 counter value  WDTSPGM=WDT stops during Flash programming  FDMTEN=Deadman Timer is disabled  TRCEN=Trace features in the CPU are enabled  BOOTISA=Boot code and Exception code is MIPS32  FECCCON=ECC and Dynamic ECC are disabled (ECCCON bits are writable)  EXTDDRSIZE=Not used  FSLEEP=Flash is powered down when the device is in Sleep mode  DBGPER=Allow CPU access to all permission regions  EJTAGBEN=Normal EJTAG functionality  TSEQ=Not used  CSEQ=Not used  RWDTPS=1:1048576  RCLKSEL=Always use LPRC  SWDTPS=1:1048576  DMTIVTL=Not used  DMTIVTH=Not used  DMTCNTL=Not used  DMTCNTH=Not used  DMTDIS=Dead Man Timer is Disabled and can be enabled by software  SMBEN=SMBus input threshold is enabled  SPI2PIN=SPI2 uses I/O remap (PPS) pins  CTXT3=Not Assigned  CTXT4=Not Assigned  MBXM0=Mailbox register configured for Main data read (Secondary to Main data transfer)  MBXM1=Mailbox register configured for Main data read (Secondary to Main data transfer)  MBXM2=Mailbox register configured for Main data read (Secondary to Main data transfer)  MBXM3=Mailbox register configured for Main data read (Secondary to Main data transfer)  MBXM4=Mailbox register configured for Main data read (Secondary to Main data transfer)  MBXM5=Mailbox register configured for Main data read (Secondary to Main data transfer)  MBXM6=Mailbox register configured for Main data read (Secondary to Main data transfer)  MBXM7=Mailbox register configured for Main data read (Secondary to Main data transfer)  MBXM8=Mailbox register configured for Main data read (Secondary to Main data transfer)  MBXM9=Mailbox register configured for Main data read (Secondary to Main data transfer)  MBXM10=Mailbox register configured for Main data read (Secondary to Main data transfer)  MBXM11=Mailbox register configured for Main data read (Secondary to Main data transfer)  MBXM12=Mailbox register configured for Main data read (Secondary to Main data transfer)  MBXM13=Mailbox register configured for Main data read (Secondary to Main data transfer)  MBXM14=Mailbox register configured for Main data read (Secondary to Main data transfer)  MBXM15=Mailbox register configured for Main data read (Secondary to Main data transfer)  MBXHSA=MSIxMBXD15 assigned to mailbox handshake protocol block A  MBXHSB=MSIxMBXD15 assigned to mailbox handshake protocol block B  MBXHSC=MSIxMBXD15 assigned to mailbox handshake protocol block C  MBXHSD=MSIxMBXD15 assigned to mailbox handshake protocol block D  MBXHSE=MSIxMBXD15 assigned to mailbox handshake protocol block E  MBXHSF=MSIxMBXD15 assigned to mailbox handshake protocol block F  MBXHSG=MSIxMBXD15 assigned to mailbox handshake protocol block G  MBXHSH=MSIxMBXD15 assigned to mailbox handshake protocol block H  HSAEN=Mailbox data flow control handshake protocol block disabled  HSBEN=Mailbox data flow control handshake protocol block disabled  HSCEN=Mailbox data flow control handshake protocol block disabled  HSDEN=Mailbox data flow control handshake protocol block disabled  HSEEN=Mailbox data flow control handshake protocol block disabled  HSFEN=Mailbox data flow control handshake protocol block disabled  HSGEN=Mailbox data flow control handshake protocol block disabled  HSHEN=Mailbox data flow control handshake protocol block disabled  CPRA0=Main core owns pin  CPRA1=Main core owns pin  CPRA2=Main core owns pin  CPRA3=Main core owns pin  CPRA4=Main core owns pin  CPRB0=Main core owns pin  CPRB1=Main core owns pin  CPRB2=Main core owns pin  CPRB3=Main core owns pin  CPRB4=Main core owns pin  CPRB5=Main core owns pin  CPRB6=Main core owns pin  CPRB7=Main core owns pin  CPRB8=Main core owns pin  CPRB9=Main core owns pin  CPRB10=Main core owns pin  CPRB11=Main core owns pin  CPRB12=Main core owns pin  CPRB13=Main core owns pin  CPRB14=Main core owns pin  CPRB15=Main core owns pin  CPRC0=Main core owns pin  CPRC1=Main core owns pin  CPRC2=Main core owns pin  CPRC3=Main core owns pin  CPRC4=Main core owns pin  CPRC5=Main core owns pin  CPRC6=Main core owns pin  CPRC7=Main core owns pin  CPRC8=Main core owns pin  CPRC9=Main core owns pin  CPRC10=Main core owns pin  CPRC11=Main core owns pin  CPRC12=Main core owns pin  CPRC13=Main core owns pin  CPRC14=Main core owns pin  CPRC15=Main core owns pin  CPRD0=Main core owns pin  CPRD1=Main core owns pin  CPRD2=Main core owns pin  CPRD3=Main core owns pin  CPRD4=Main core owns pin  CPRD5=Main core owns pin  CPRD6=Main core owns pin  CPRD7=Main core owns pin  CPRD8=Main core owns pin  CPRD9=Main core owns pin  CPRD10=Main core owns pin  CPRD11=Main core owns pin  CPRD12=Main core owns pin  CPRD13=Main core owns pin  CPRD14=Main core owns pin  CPRD15=Main core owns pin  CPRE0=Main core owns pin  CPRE1=Main core owns pin  CPRE2=Main core owns pin  CPRE3=Main core owns pin  CPRE4=Main core owns pin  CPRE5=Main core owns pin  CPRE6=Main core owns pin  CPRE7=Main core owns pin  CPRE8=Main core owns pin  CPRE9=Main core owns pin  CPRE10=Main core owns pin  CPRE11=Main core owns pin  CPRE12=Main core owns pin  CPRE13=Main core owns pin  CPRE14=Main core owns pin  CPRE15=Main core owns pin  S1FNOSC=Internal Fast RC (FRC) Oscillator with postscaler  S1IESO=Start up with FRC; then switch  S1OSCIOFNC=OSC2 is clock output  S1FCKSM=Both Clock switching and Fail-safe Clock Monitor are disabled  S1PLLKEN=S1PLLKEN_ON  S1RWDTPS=1:1048576  S1RCLKSEL=Always use LPRC  S1WINDIS=Watchdog Timer operates in Non-Window mode  S1WDTWIN=WDT Window is 25% of WDT period  S1SWDTPS=1:1048576  S1FWDTEN=use WDTCON.ON bit  S1ICS=Communicate on PGC3 and PGD3  S1DEBUG=Not used  S1ISOLAT=The Secondary can operate (in debug mode) even if the SLVEN bit in the MSI is zero  S1NOBTSWP=BOOTSWP instruction is disabled  S1ALTI2C1=I2C1 mapped to SDA1/SCL1 pins  S1SPI1PIN=Secondary SPI1 uses I/O remap (PPS) pins  S1SSRE=Secondary generated resets will reset the Secondary Enable Bit in the MSI module  S1MSRE=The Main software oriented RESET events (RESET Op-Code; Watchdog timeout; TRAP reset; illegalInstruction) will also cause the Secondary subsystem to reset  S1CTXT1=Not Assigned  S1CTXT2=Not Assigned  S1CTXT3=Not Assigned  S1CTXT4=Not Assigned  BORLVL=Not used  BSSO=Not used  MCA=Not used  MAXTEMP=Not used  CFGAN14=Not used  CFGAN15=Not used  S1IOL1WAY=Not used  S1BSSO=Not used  S1BACKBUG=Not used  BISTDIS=mBIST on reset feature disabled  NOBTSWP=BOOTSWP instruction is disabled  S1BISTDIS=Secondary BIST on reset feature disabled  S1DMTIVTL=Not used  S1DMTIVTH=Not used  S1DMTCNTL=Not used  S1DMTCNTH=Not used  S1DMTDIS=Secondary Dead Man Timer is Disabled and can be enabled by software  BSEQ=Not used  IBSEQ=Not used  SMB3EN=SMBus 3.0 input levels  FUSBIDIO2=USBID pin is controlled by the USB2 module  FVBUSIO2=VBUSON pin is controlled by the USB2 module  FUSBIDIO1=USBID pin is controlled by the USB1 module  FVBUSIO1=VBUSON pin is controlled by the USB1 module  VBATBOREN=Enable ZPBOR during VBAT Mode  FDSEN=Enable DSEN bit in DSCON  BORSEL=BOR trip voltage 2.1v (Non-OPAMP deviced operation)  POSCFGAIN=Gain is G3  POSCAGCDLY=Settling time = 25ms x AGCRNG  POSCAGCRNG=Range 1x  POSCAGC=Automatic Gain Control for Oscillator  FDBGWP=Not used
  PIM  LED RED : MCHP_Blockset/Digital IO/Digital Output Write  PORT=Dynamic Options  PORT_TXT="B   [ 0 : 11 ]"  PIN=0  INIT_VALUE=-1  PACK=off  OUTPUT_PIN_MODE=Push-Pull (default)  SIMULTANEOUS=off  ORDERING=None  SampleTime=-1  MCHP_PORT={Digital Out}{DOU}1:1:B0;  MCHP_MASTERLINK=dsPIC33AK512MPS506_DPDB_External_v4/Microchip Master
  PWM_HS_FEP : MCHP_Blockset/PWM IO/PWM_HS_FEP  Priority=-2000  PWMx_MODSEL=Edge Aligned - Duty Cycle and Phase Shift  PWMx_CLKSEL=Use divider circuit  PWM_ClockResolution_DIVSEL=Dynamic Options  PWM_ClockResolution_DIVSEL_TXT=auto  PWM_ClockResolution_FSCL=Dynamic Options  PWM_ClockResolution_FSCL_TXT="Resol: 0.05(us)  -  MaxPer: 0.00328(s)"  PWM_ClockResolution_NoScaling=Dynamic Options  PWM_ClockResolution_NoScaling_TXT="Resol: 0.005(us)  -  MaxPer: 0.000328(s)"  MaxPeriod_s=10e-6  InitPeriode_s=10e-6  InitDutyCycleP_s=0  InitDutyCycleS_s=10e-6  InitPhase_s=-1  evalin_ws=PWM1max=MCHP_Fun.Hex2num('409F400000000001');PWM2max=MCHP_Fun.Hex2num('409F400000000001');  SampleTime=-1  S_INPUT=[-1]  S_INPUT_Size=[3]  S_OUTPUT=[]  S_OUTPUT_Size=[]  S_ListCustomDatatype=S.S_ListCustomDatatype={};  MCHP_USER_INTERRUPTS=0  MCHP_PORT={PWMH1 }{PWMH1}32:4:D2;{PWMH2 }{PWMH2}32:4:D0;{PWML1}{PWML1}32:4:D3;{PWML2}{PWML2}32:4:D1;  MCHP_MASTERLINK=dsPIC33AK512MPS506_DPDB_External_v5/Microchip Master  MCHP_CRC=4755063  PWMx_PMOD=Complementary  PWM1_HL=PWMxH & PWMxL output enabled  PWM1_swap=off  PWM1H_pol=off  PWM1L_pol=off  PWM2_HL=PWMxH & PWMxL output enabled  PWM2_swap=off  PWM2H_pol=off  PWM2L_pol=off  PWM3_HL=not used  PWM3_swap=off  PWM3H_pol=off  PWM3L_pol=off  PWM4_HL=not used  PWM4_swap=off  PWM4H_pol=off  PWM4L_pol=off  PWM5_HL=not used  PWM5_swap=off  PWM5H_pol=off  PWM5L_pol=off  PWM6_HL=not used  PWM6_swap=off  PWM6H_pol=off  PWM6L_pol=off  PWM7_HL=not used  PWM7_swap=off  PWM7H_pol=off  PWM7L_pol=off  PWM8_HL=not used  PWM8_swap=off  PWM8H_pol=off  PWM8L_pol=off  PWM9_HL=not used  PWM9_swap=off  PWM9H_pol=off  PWM9L_pol=off  PWM10_HL=not used  PWM10_swap=off  PWM10H_pol=off  PWM10L_pol=off  PWM11_HL=not used  PWM11_swap=off  PWM11H_pol=off  PWM11L_pol=off  PWM12_HL=not used  PWM12_swap=off  PWM12H_pol=off  PWM12L_pol=off  PWM1_ShowTrig=on  PWM1_Init_PGxTRIGABC_s=[0 -1 -1 ]  PWM1_ADTRxEN1=ADC Trigger 1  PWM1_ADTRxEN2=none  PWM1_ADTRxEN3=none  PWM2_ShowTrig=on  PWM2_Init_PGxTRIGABC_s=[-1 -1 -1]  PWM2_ADTRxEN1=none  PWM2_ADTRxEN2=none  PWM2_ADTRxEN3=none  PWM3_ShowTrig=off  PWM3_Init_PGxTRIGABC_s=[-1 -1 -1]  PWM3_ADTRxEN1=none  PWM3_ADTRxEN2=none  PWM3_ADTRxEN3=none  PWM4_ShowTrig=off  PWM4_Init_PGxTRIGABC_s=[-1 -1 -1]  PWM4_ADTRxEN1=none  PWM4_ADTRxEN2=none  PWM4_ADTRxEN3=none  PWM5_ShowTrig=off  PWM5_Init_PGxTRIGABC_s=[-1 -1 -1]  PWM5_ADTRxEN1=none  PWM5_ADTRxEN2=none  PWM5_ADTRxEN3=none  PWM6_ShowTrig=off  PWM6_Init_PGxTRIGABC_s=[-1 -1 -1]  PWM6_ADTRxEN1=none  PWM6_ADTRxEN2=none  PWM6_ADTRxEN3=none  PWM7_ShowTrig=off  PWM7_Init_PGxTRIGABC_s=[-1 -1 -1]  PWM7_ADTRxEN1=none  PWM7_ADTRxEN2=none  PWM7_ADTRxEN3=none  PWM8_ShowTrig=off  PWM8_Init_PGxTRIGABC_s=[-1 -1 -1]  PWM8_ADTRxEN1=none  PWM8_ADTRxEN2=none  PWM8_ADTRxEN3=none  BlockInput_VectorScalar=Independant Scalar  BlockInput_Period=Not a block input  BlockInput_DutyCycle=a Floating Point input within range [0 1]  BlockInput_PhaseShift=Not a block input  BlockInput_SEVTCMP=Not a block input  BlockInput_TRIGx=Not a block input  BlockInput_DeadTime=Not a block input  BlockOutput_FaultDisabled=off  BlockOutput_Fault=on  DTC=Positive dead time (ensure period of time with PWM_H and PWM_L disasserted)  FLTSRC1_DTCMP=Dynamic Options  FLTSRC1_DTCMP_TXT=<empty>  FLTSRC2_DTCMP=Dynamic Options  FLTSRC2_DTCMP_TXT=<empty>  FLTSRC3_DTCMP=Dynamic Options  FLTSRC3_DTCMP_TXT=<empty>  FLTSRC4_DTCMP=Dynamic Options  FLTSRC4_DTCMP_TXT=<empty>  FLTSRC5_DTCMP=Dynamic Options  FLTSRC5_DTCMP_TXT=<empty>  FLTSRC6_DTCMP=Dynamic Options  FLTSRC6_DTCMP_TXT=<empty>  FLTSRC7_DTCMP=Dynamic Options  FLTSRC7_DTCMP_TXT=<empty>  FLTSRC8_DTCMP=Dynamic Options  FLTSRC8_DTCMP_TXT=<empty>  FLTSRC9_DTCMP=Dynamic Options  FLTSRC9_DTCMP_TXT=<empty>  FLTSRC10_DTCMP=Dynamic Options  FLTSRC10_DTCMP_TXT=<empty>  FLTSRC11_DTCMP=Dynamic Options  FLTSRC11_DTCMP_TXT=<empty>  FLTSRC12_DTCMP=Dynamic Options  FLTSRC12_DTCMP_TXT=<empty>  DeadTime_s=2e-6  DeadTimeAlt_s=2e-6  DeadTimeComp_s=0  FLTMODx=Disabled  FLTSRCx=Dynamic Options  FLTSRCx_TXT=<empty>  FLTDATx=PWM H/L -> 11  CLMODx=Disabled  CLSRCx=Dynamic Options  CLSRCx_TXT=<empty>  CLDATx=PWM H/L -> 00  FLTLEBENx=off  CLLEBENx=off  LeadEdgeBlkPer_s=5e-7  PHRx=off  PHFx=off  PLRx=off  PLFx=off
  Port Info : MCHP_Blockset/System Info/Port Info  MCHP_MASTERLINK=dsPIC33AK512MPS506_DPDB_External_v4/Microchip Master
  Rate Transition{,1..3} (4 alike) : RateTransition  OutPortSampleTime=.001
  Scope : Scope
  Scope1 : Scope  NumInputPorts=2
  SinCos1 : Trigonometry  AngleUnit=revolution  TableDataTypeStr=fixdt(1,16,15)
  Slider : SliderBlock  ScaleMin=0.1  ScaleMax=20
  Sum1 : Sum  Inputs=|++
  Terminator : Terminator
  Timer Info : MCHP_Blockset/System Info/Timer Info  MCHP_MASTERLINK=dsPIC33AK512MPS506_DPDB_External_v4/Microchip Master
  UART configuration DEBUG JP4-JP5 : MCHP_Blockset/BUS UART/UART Configuration  UART_REF=1  BAUD_Choice=Dynamic Options  BAUD_Choice_TXT="460800         [+0.01%]"  BAUD_Choice_IR=Dynamic Options  BAUD_Choice_IR_TXT=[]  BAUD_Custom=115200  INT_PRIORITY=0  ALT_IO=on  PIN_RX=Dynamic Options  PIN_RX_TXT=C6 / P39 / Pin[35]  PIN_RX_INPUT_MODE=Hi-impedance (default)  PIN_TX=Dynamic Options  PIN_TX_TXT=C7 / P40 / Pin[36]  PIN_TX_OUTPUT_MODE=Push-Pull (default)  MCHP_PORT="{UART1  Rx}{U1RX}3:0:P39;{UART1  Tx}{U1TX}3:0:P40;"  MCHP_MASTERLINK=dsPIC33AK512MPS506_DPDB_External_v4/Microchip Master  MCHP_COM_ExtPil=on  TX_IMPLEMENTATION=Circular Buffer  TX_IMPLEMENTATION_default=Circular Buffer  TX_INT_PRIORITY=5  TX_INT_WHEN=is empty & last char is sent  TX_INT_WHEN_default=is empty & last char is sent  TX_CIRCULAR_SIZE=256  TX_DMA_CHANNEL="0   (Lowest Priority)"  TX_DMA_SIZE=512  TX_TASK_PROTECTION=Delay tasks (default)  TX_INTERRUPT_PROTECTION=Do not send on conflict (default)  TX_INTERRUPT_PROTECTION_default=Do not send on conflict (default)  RX_IMPLEMENTATION=Circular Buffer  RX_IMPLEMENTATION_default=Circular Buffer  RX_INT_PRIORITY=5  RX_INT_WHEN=is 3/4 fulll (contains 3 data characters)  RX_CIRCULAR_SIZE=64  RX_DMA_CHANNEL=0  RX_DMA_SIZE=0  DuplexMode=Full duplex (default)  PIN_RX_Inv=off  PIN_TX_Inv=off  PIN_RXTX_Inv=off  ParityBit=No parity (default)  StopBit=1 stop bit (default)  IRDA=off  IdleTime_choice=Dynamic Options  IdleTime_choice_TXT=None  IdleTime_custom=2/50  FlowControl=None  PIN_CTS=Dynamic Options  PIN_CTS_TXT=B0 / P17 / Pin[20]  PIN_CTS_INPUT_MODE=Hi-impedance (default)  PIN_RTS=Dynamic Options  PIN_RTS_TXT=B0 / P17 / Pin[20]  PIN_RTS_OUTPUT_MODE=Push-Pull (default)  PIN_DSR=Dynamic Options  PIN_DSR_TXT=B0 / P17 / Pin[20]  PIN_DSR_INPUT_MODE=Hi-impedance (default)  PIN_DTR=Dynamic Options  PIN_DTR_TXT=B0 / P17 / Pin[20]  PIN_DTR_OUTPUT_MODE=Push-Pull (default)  InitSequence_chkbox=off  BAUD_Choice_InitSeq=Dynamic Options  BAUD_Choice_InitSeq_TXT="115200         [+0.01%]"  BAUD_Choice_IR_InitSeq=Dynamic Options  BAUD_Choice_IR_InitSeq_TXT=0  BAUD_Custom_InitSeq=0  InitSequence="uint8(['use VT100 terminal ! ' 13 10 27 'c'  27 '[2J' ] )"
  Weighted Sample Time : SampleTimeMath  TsampMathOp=*  weightValue=1  OutDataTypeStr=fixdt(0,32,32)  RndMeth=Round  SaturateOnIntegerOverflow=on
  dsPIC 33AK512MPS506 PIM Webpage : Subsystem
  frequency1 : Constant  Value=3.057275541795665  OutDataTypeStr=fixdt(0,16,8)  SampleTime=0.1
  frequency2 : Constant  Value=4  OutDataTypeStr=fixdt(0,16,8)  SampleTime=0.1
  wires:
  Heart beat/1 -> Cast/1
  Cast/1 -> PIM  LED RED/1
  Cast4/1 -> Gain/1
  Sum1/1 -> Delay1/1
  frequency1/1 -> Manual Switch/2
  Delay1/1 -> Cast4/1, Sum1/2
  Weighted Sample Time/1 -> Sum1/1
  SinCos1/1 -> PWM_HS_FEP/2, Scope/1  "SineU1 CH3"
  MCU Load/1 -> MCU load/1
  MCU load/1 -> Display/1
  Rate Transition/1 -> Weighted Sample Time/1
  Manual Switch/1 -> Rate Transition/1
  frequency2/1 -> Manual Switch/1
  ADC HS 12b dsPICA/1 -> Rate Transition1/1
  ADC HS 12b dsPICA/2 -> Gain1/1, Rate Transition2/1
  Gain/1 -> SinCos1/1  "Angle"
  Gain1/1 -> Rate Transition3/1, Cast3/1
  Cast3/1 -> PWM_HS_FEP/1
  Rate Transition1/1 -> Scope1/1  "AD2"
  Rate Transition2/1 -> Scope1/2  "AD5"
  Rate Transition3/1 -> Terminator/1  "AD5_scaled"
